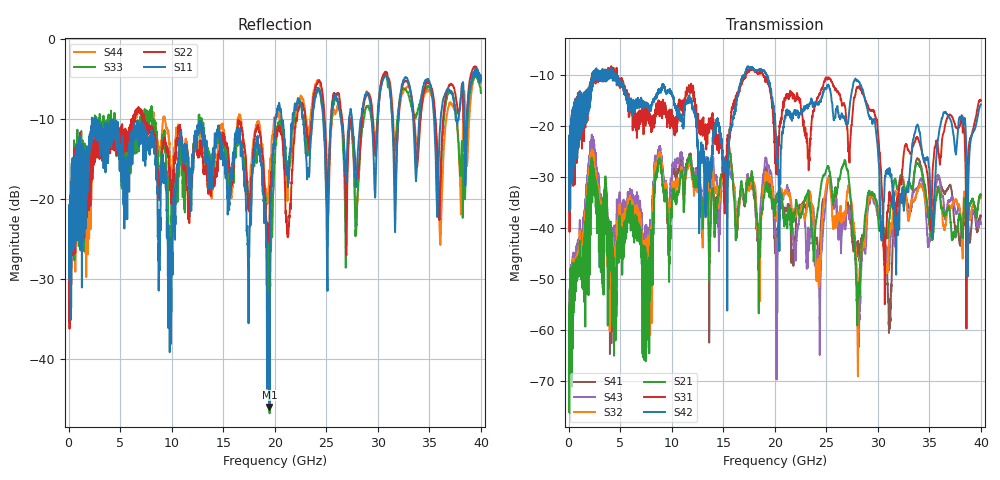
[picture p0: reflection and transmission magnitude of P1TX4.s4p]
!Agilent Technologies,N5245A,MY49151084,A.09.20.08
!Agilent N5245A: A.09.20.08
!Date: Thursday, March 01, 2012 13:56:01
!Correction: S11(Full 4 Port(1,2,3,4))
!S12(Full 4 Port(1,2,3,4))
!S13(Full 4 Port(1,2,3,4))
!S14(Full 4 Port(1,2,3,4))
!S21(Full 4 Port(1,2,3,4))
!S22(Full 4 Port(1,2,3,4))
!S23(Full 4 Port(1,2,3,4))
!S24(Full 4 Port(1,2,3,4))
!S31(Full 4 Port(1,2,3,4))
!S32(Full 4 Port(1,2,3,4))
!S33(Full 4 Port(1,2,3,4))
!S34(Full 4 Port(1,2,3,4))
!S41(Full 4 Port(1,2,3,4))
!S42(Full 4 Port(1,2,3,4))
!S43(Full 4 Port(1,2,3,4))
!S44(Full 4 Port(1,2,3,4))
!S4P File: Measurements: <S11,S12,S13,S14>,
!<S21,S22,S23,S24>,
!<S31,S32,S33,S34>,
!<S41,S42,S43,S44>:
# Hz S  dB  R 50
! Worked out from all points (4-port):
!   3996 points, 50 MHz to 40 GHz, reference 50 ohm
!   strongest paths, dB at 50 MHz, 10.04 GHz, 20.03 GHz, 30.02 GHz, 40 GHz:
!     S42: -24.7, -13.8, -19.0, -25.1, -15.8
!     S31: -26.3, -18.8, -26.6, -21.3, -15.1
!     S21: -58.9, -34.7, -37.7, -37.8, -33.6
!     S32: -63.6, -33.0, -37.6, -36.5, -34.2
!     S43: -57.5, -29.0, -40.6, -37.8, -39.2
!     S41: -58.1, -30.0, -44.1, -36.0, -37.8
!   lowest |S11| = -45.9 dB at 19.49 GHz (marker M1), VSWR 1.01, Z = 50.3 - j0.412 ohm
!   |S11| at or under -10 dB: start of sweep to 2.258 GHz; 2.621 GHz to 20.05 GHz (17.42 GHz wide, 154 % of centre); 20.66 GHz to 21.73 GHz (1.064 GHz wide, 5.02 % of centre)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
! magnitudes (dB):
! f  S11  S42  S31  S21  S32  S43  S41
! 50 MHz  -24.5  -24.7  -26.3  -58.9  -63.6  -57.5  -58.1
! 2.32 GHz  -11.0  -12.3  -10.6  -28.8  -26.1  -22.6  -25.1
! 4.48 GHz  -11.8  -11.2  -9.7  -55.6  -44.9  -41.4  -47.4
! 19.49 GHz  -45.9  -11.9  -12.1  -34.0  -30.9  -29.5  -32.1
! 28.26 GHz  -10.7  -11.7  -12.6  -51.5  -48.1  -55.9  -47.3
! 30.69 GHz  -4.7  -30.1  -52.0  -41.1  -46.8  -45.5  -44.5
! 40 GHz  -5.3  -15.8  -15.1  -33.6  -34.2  -39.2  -37.8
